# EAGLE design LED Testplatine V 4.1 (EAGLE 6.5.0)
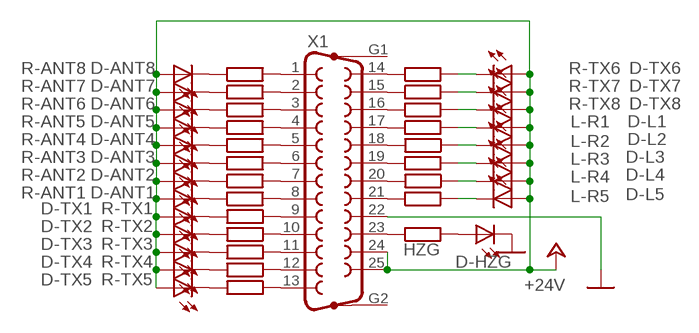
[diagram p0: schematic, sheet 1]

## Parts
D-ANT1  LEDCHIPLED_1206  [CHIPLED_1206]
D-ANT2  LEDCHIPLED_1206  [CHIPLED_1206]
D-ANT3  LEDCHIPLED_1206  [CHIPLED_1206]
D-ANT4  LEDCHIPLED_1206  [CHIPLED_1206]
D-ANT5  LEDCHIPLED_1206  [CHIPLED_1206]
D-ANT6  LEDCHIPLED_1206  [CHIPLED_1206]
D-ANT7  LEDCHIPLED_1206  [CHIPLED_1206]
D-ANT8  LEDCHIPLED_1206  [CHIPLED_1206]
D-HZG  LEDCHIPLED_1206  [CHIPLED_1206]
D-L1  LEDCHIPLED_1206  [CHIPLED_1206]
D-L2  LEDCHIPLED_1206  [CHIPLED_1206]
D-L3  LEDCHIPLED_1206  [CHIPLED_1206]
D-L4  LEDCHIPLED_1206  [CHIPLED_1206]
D-L5  LEDCHIPLED_1206  [CHIPLED_1206]
D-TX1  LEDCHIPLED_1206  [CHIPLED_1206]
D-TX2  LEDCHIPLED_1206  [CHIPLED_1206]
D-TX3  LEDCHIPLED_1206  [CHIPLED_1206]
D-TX4  LEDCHIPLED_1206  [CHIPLED_1206]
D-TX5  LEDCHIPLED_1206  [CHIPLED_1206]
D-TX6  LEDCHIPLED_1206  [CHIPLED_1206]
D-TX7  LEDCHIPLED_1206  [CHIPLED_1206]
D-TX8  LEDCHIPLED_1206  [CHIPLED_1206]
HZG  R-EU_R1206  [R1206]
L-R1  R-EU_R1206  [R1206]
L-R2  R-EU_R1206  [R1206]
L-R3  R-EU_R1206  [R1206]
L-R4  R-EU_R1206  [R1206]
L-R5  R-EU_R1206  [R1206]
R-ANT1  R-EU_R1206  [R1206]
R-ANT2  R-EU_R1206  [R1206]
R-ANT3  R-EU_R1206  [R1206]
R-ANT4  R-EU_R1206  [R1206]
R-ANT5  R-EU_R1206  [R1206]
R-ANT6  R-EU_R1206  [R1206]
R-ANT7  R-EU_R1206  [R1206]
R-ANT8  R-EU_R1206  [R1206]
R-TX1  R-EU_R1206  [R1206]
R-TX2  R-EU_R1206  [R1206]
R-TX3  R-EU_R1206  [R1206]
R-TX4  R-EU_R1206  [R1206]
R-TX5  R-EU_R1206  [R1206]
R-TX6  R-EU_R1206  [R1206]
R-TX7  R-EU_R1206  [R1206]
R-TX8  R-EU_R1206  [R1206]
X1  F25HP  [F25HP]

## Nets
+24V: D-ANT1.A D-ANT2.A D-ANT3.A D-ANT4.A D-ANT5.A D-ANT6.A D-ANT7.A D-ANT8.A D-L1.A D-L2.A D-L3.A D-L4.A D-L5.A D-TX1.A D-TX2.A D-TX3.A D-TX4.A D-TX5.A D-TX6.A D-TX7.A D-TX8.A X1.24 X1.25
GND: D-HZG.C X1.22
N$1: R-TX1.1 X1.9
N$2: R-TX2.1 X1.10
N$3: R-TX3.1 X1.11
N$4: R-TX4.1 X1.12
N$5: R-TX5.1 X1.13
N$6: L-R1.1 X1.17
N$7: R-TX6.1 X1.14
N$8: R-TX7.1 X1.15
N$9: R-TX8.1 X1.16
N$10: L-R2.2 X1.18
N$11: L-R3.1 X1.19
N$12: L-R4.2 X1.20
N$13: R-ANT8.2 X1.1
N$14: R-ANT7.2 X1.2
N$15: R-ANT6.2 X1.3
N$16: R-ANT5.2 X1.4
N$17: R-ANT4.2 X1.5
N$18: R-ANT3.2 X1.6
N$19: R-ANT2.2 X1.7
N$20: R-ANT1.2 X1.8
N$21: L-R5.1 X1.21
N$23: D-HZG.A HZG.2
N$24: D-L1.C L-R1.2
N$25: D-L3.C L-R3.2
N$26: D-L5.C L-R5.2
N$27: HZG.1 X1.23
N$28: D-L2.C L-R2.1
N$29: D-L4.C L-R4.1
N$31: D-TX1.C R-TX1.2
N$32: D-TX2.C R-TX2.2
N$33: D-TX3.C R-TX3.2
N$34: D-TX4.C R-TX4.2
N$35: D-ANT1.C R-ANT1.1
N$36: D-ANT2.C R-ANT2.1
N$37: D-ANT3.C R-ANT3.1
N$38: D-ANT4.C R-ANT4.1
N$39: D-TX5.C R-TX5.2
N$40: D-TX6.C R-TX6.2
N$41: D-TX7.C R-TX7.2
N$42: D-TX8.C R-TX8.2
N$43: D-ANT5.C R-ANT5.1
N$44: D-ANT6.C R-ANT6.1
N$45: D-ANT7.C R-ANT7.1
N$46: D-ANT8.C R-ANT8.1
Unconnected: X1.G1 X1.G2

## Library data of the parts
D-ANT1-D-ANT8 D-HZG D-L1-D-L5 D-TX1-D-TX8 = led:LED: LED
HZG L-R1-L-R5 R-ANT1-R-ANT8 R-TX1-R-TX8 = rcl:R-EU_: RESISTOR, European symbol
X1 = con-subd:F25HP: SUB-D; OC_FARNELL: unknown; OC_NEWARK: unknown

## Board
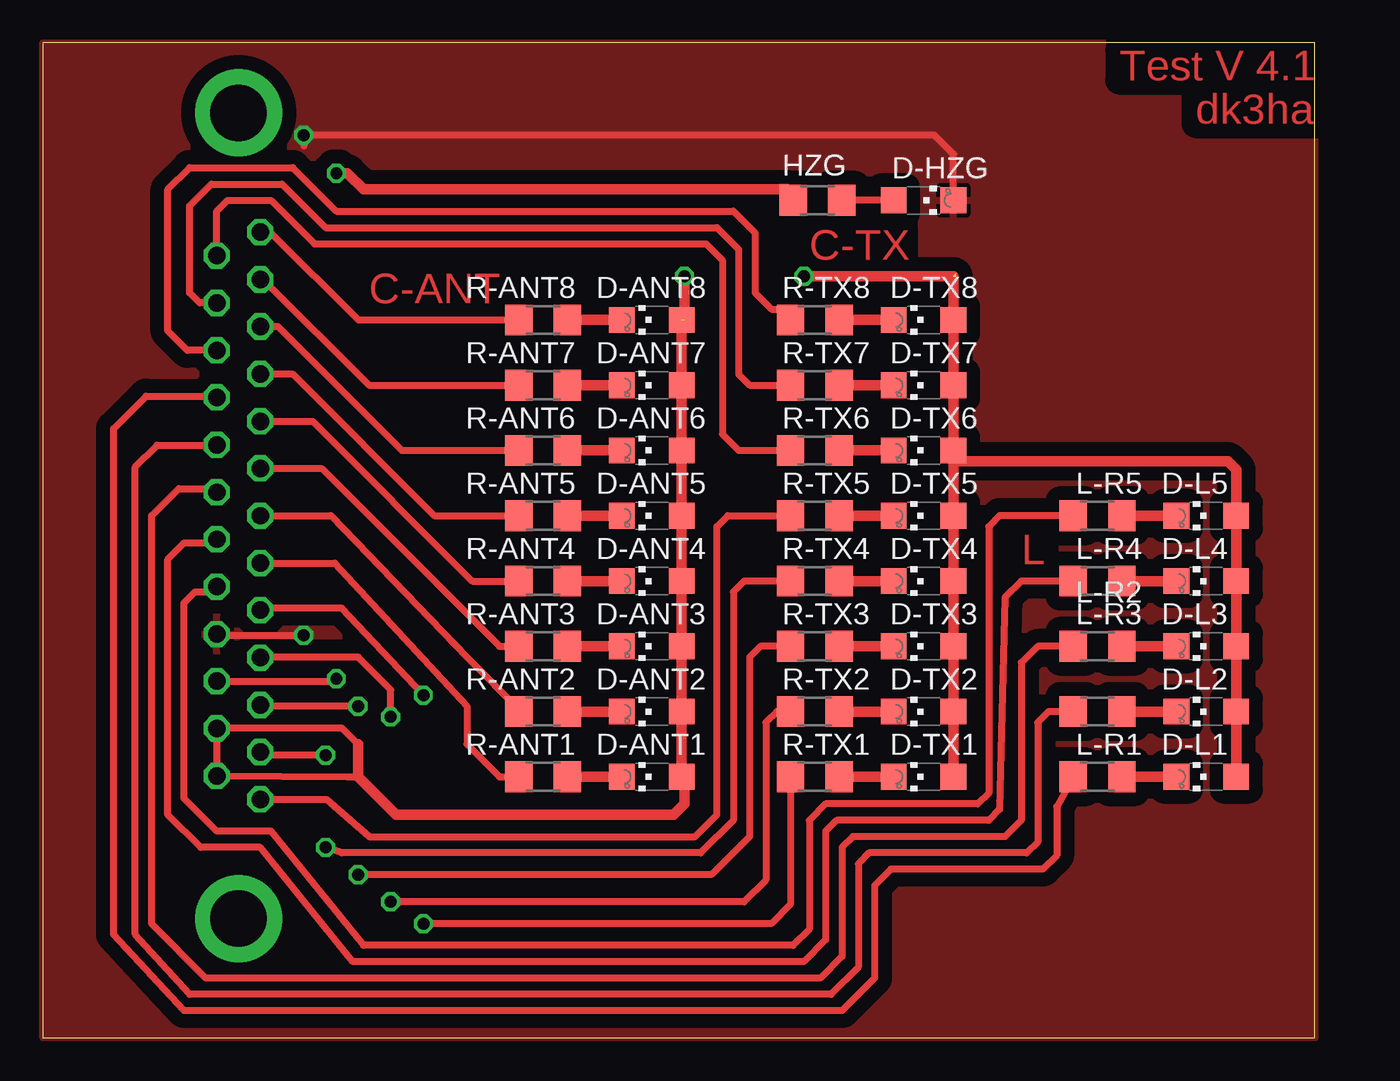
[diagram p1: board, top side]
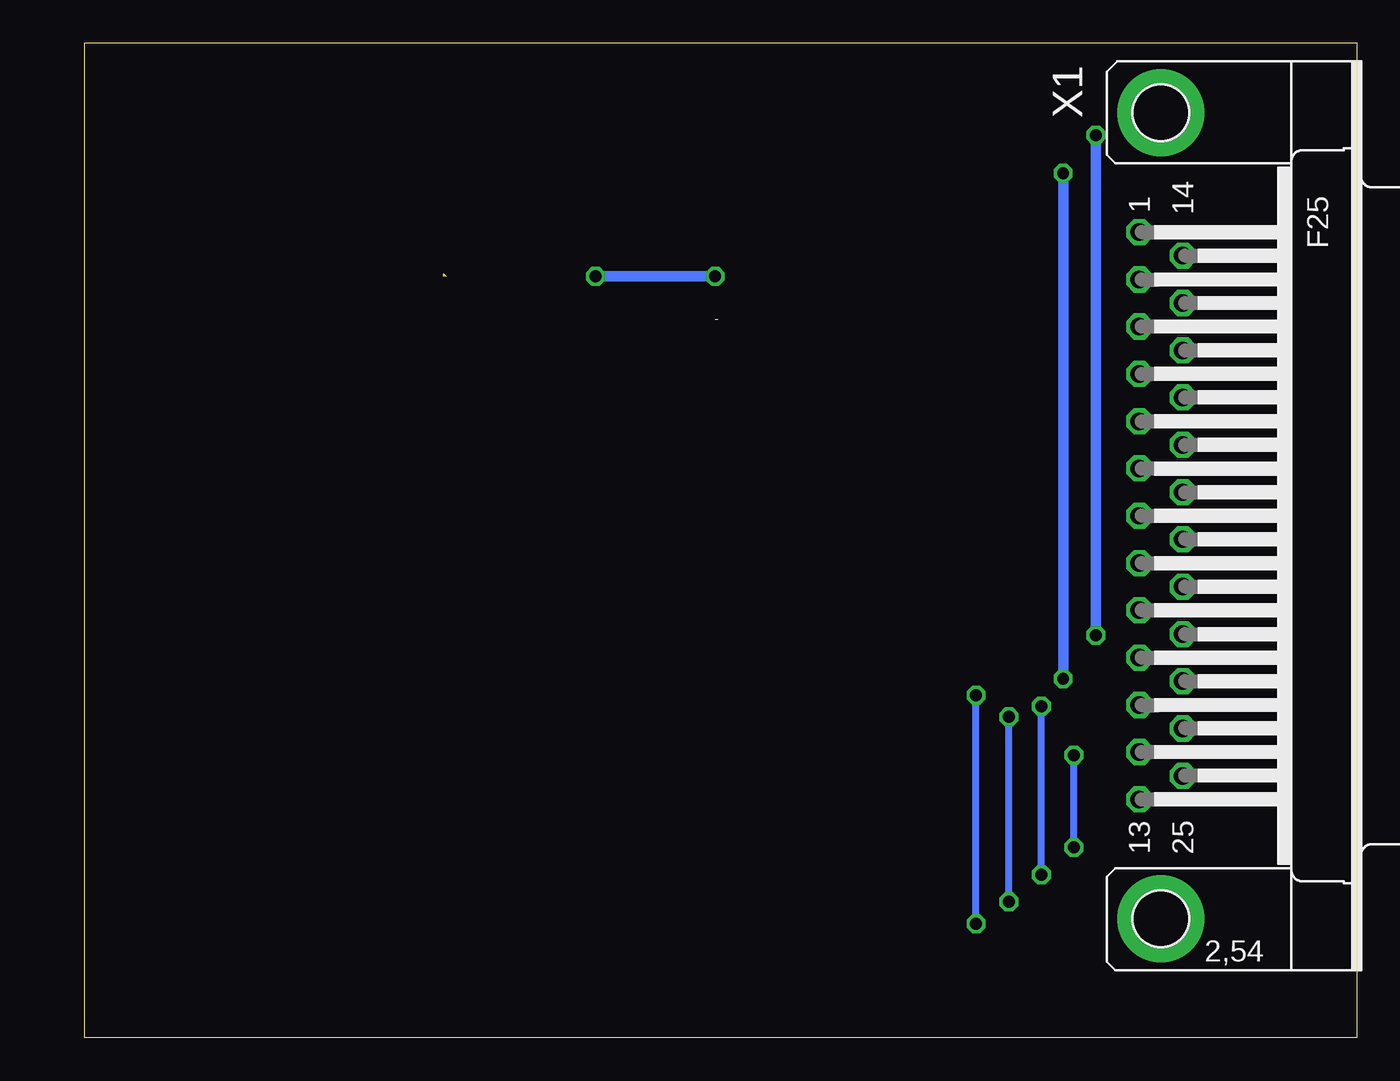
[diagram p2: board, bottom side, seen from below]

Size 74.28 x 58.09 mm. Coordinates in mm from the lower left corner, seen from the top.
Outline: 0,0 74.28,0 74.28,58.09 0,58.09 0,0
Copper layers (1*16): Top 0.035mm / dielectric 1.5mm / Bottom 0.035mm
Design rules "default *": minimum track width 10mil, minimum drill 24mil, track to track 8mil, track to pad 8mil, pad to pad 8mil, via to via 8mil, smd to smd 8mil, copper to edge 0mil, drill to drill 8mil, minimum pad ring 10mil, minimum via ring 8mil, stop-mask expansion 4mil, vias tented up to drill 0mil, thermal gap 10mil

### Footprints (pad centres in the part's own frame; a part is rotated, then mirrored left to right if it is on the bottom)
CHIPLED_1206 = smd 1.5 x 1.5: A 0,-1.75; C 0,1.75
R1206 = smd 1.6 x 1.803: 1 -1.422,0; 2 1.422,0
F25HP = drill 1.016 octagon: 1 -16.561,-1.27; 2 -13.792,-1.27; 3 -11.049,-1.27; 4 -8.28,-1.27; 5 -5.512,-1.27; 6 -2.769,-1.27; 7 0,-1.27; 8 2.769,-1.27; 9 5.512,-1.27; 10 8.28,-1.27; 11 11.049,-1.27; 12 13.792,-1.27; 13 16.561,-1.27; 14 -15.189,1.27; 15 -12.421,1.27; 16 -9.652,1.27; 17 -6.909,1.27; 18 -4.14,1.27; 19 -1.372,1.27; 20 1.372,1.27; 21 4.14,1.27; 22 6.909,1.27; 23 9.652,1.27; 24 12.421,1.27; 25 15.189,1.27 | drill 3.302 pad 5.08: G1 -23.52,0; G2 23.52,0

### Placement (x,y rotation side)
D-ANT1  35.56,15.24 90 top
D-ANT2  35.56,19.05 90 top
D-ANT3  35.56,22.86 90 top
D-ANT4  35.56,26.67 90 top
D-ANT5  35.56,30.48 90 top
D-ANT6  35.56,34.29 90 top
D-ANT7  35.56,38.1 90 top
D-ANT8  35.56,41.91 90 top
D-HZG  51.44,48.9 270 top
D-L1  67.94,15.24 90 top
D-L2  67.94,19.05 90 top
D-L3  67.94,22.86 90 top
D-L4  67.94,26.67 90 top
D-L5  67.94,30.48 90 top
D-TX1  51.44,15.24 90 top
D-TX2  51.44,19.05 90 top
D-TX3  51.44,22.86 90 top
D-TX4  51.44,26.67 90 top
D-TX5  51.44,30.48 90 top
D-TX6  51.44,34.29 90 top
D-TX7  51.44,38.1 90 top
D-TX8  51.44,41.91 90 top
HZG  45.24,48.9 0 top
L-R1  61.59,15.24 0 top
L-R2  61.59,19.05 180 top
L-R3  61.59,22.86 0 top
L-R4  61.59,26.67 180 top
L-R5  61.59,30.48 0 top
R-ANT1  29.21,15.24 180 top
R-ANT2  29.21,19.05 180 top
R-ANT3  29.21,22.86 180 top
R-ANT4  29.21,26.67 180 top
R-ANT5  29.21,30.48 180 top
R-ANT6  29.21,34.29 180 top
R-ANT7  29.21,38.1 180 top
R-ANT8  29.21,41.91 180 top
R-TX1  45.09,15.24 0 top
R-TX2  45.09,19.05 0 top
R-TX3  45.09,22.86 0 top
R-TX4  45.09,26.67 0 top
R-TX5  45.09,30.48 0 top
R-TX6  45.09,34.29 0 top
R-TX7  45.09,38.1 0 top
R-TX8  45.09,41.91 0 top
X1  11.43,30.48 270 bottom

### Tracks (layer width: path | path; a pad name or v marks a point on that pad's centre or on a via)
+24V  (via drill 0.7)  (4 unrouted)
  Top 0.406: X1.24 X1.25 17.78,15.24 18.41,15.24 | 37.47,15.09 D-ANT1.A | 10.16,18.1 17.46,18.1 18.41,17.14
  Top 0.61: D-ANT8.A D-ANT7.A D-ANT6.A D-ANT5.A D-ANT4.A D-ANT3.A D-ANT2.A D-ANT1.A | 53.19,33.66 D-TX6.A D-TX7.A D-TX8.A 53.19,44.45 v44.45,44.45 | 53.19,33.66 D-TX5.A D-TX4.A D-TX3.A D-TX2.A D-TX1.A | D-L1.A D-L2.A D-L3.A D-L4.A D-L5.A 69.69,33.17 69.22,33.66 53.19,33.66 | 37.47,15.09 37.47,13.65 36.83,13.02 20.64,13.02 18.41,15.24 18.41,17.14 | 37.47,41.91 v37.47,44.45
  Bottom 0.61: v37.47,44.45 v44.45,44.45
GND  (via drill 0.7)
  Top 0.406: v15.24,23.49 10.24,23.49 X1.22 | 15.24,52.07 v15.24,52.71 52.07,52.71 53.19,51.59 D-HZG.C
  Bottom 0.61: v15.24,23.49 v15.24,52.71
  pour Top (isolate 0.813): 0,58.1 74.3,58.1 74.3,0 0,0
N$1  (via drill 0.7)
  Top 0.406: R-TX1.1 43.66,7.79 42.55,6.67 v22.23,6.67 | v22.23,20 17.46,25.08 12.81,25.08 X1.9
  Bottom 0.406: v22.23,6.67 v22.23,20
N$2  (via drill 0.7)
  Top 0.406: R-TX2.1 42.86,19.05 42.23,18.41 42.23,9.21 40.96,7.94 v20.32,7.94 | v20.32,18.73 20.32,20.32 18.41,22.22 12.72,22.22 X1.10
  Bottom 0.406: v20.32,7.94 v20.32,18.73
N$3  (via drill 0.7)
  Top 0.406: R-TX3.1 41.91,22.86 41.27,22.22 41.27,11.75 39.05,9.53 v18.41,9.53 | v18.41,19.37 12.76,19.37 X1.11
  Bottom 0.406: v18.41,9.53 v18.41,19.37
N$4  (via drill 0.7)
  Top 0.406: R-TX4.1 40.96,26.67 40.32,26.04 40.32,12.7 38.42,10.79 17.46,10.79 v16.51,11.11 | v16.51,16.51 12.88,16.51 X1.12
  Bottom 0.406: v16.51,11.11 v16.51,16.51
N$5
  Top 0.406: X1.13 16.56,13.92 19.05,11.75 38.1,11.75 39.37,13.02 39.37,29.84 40.01,30.48 R-TX5.1
N$6
  Top 0.406: L-R1.1 59.22,13.5 59.22,10.64 58.42,9.84 49.53,9.84 48.58,8.89 48.58,3.49 46.67,1.59 8.26,1.59 4.13,6.03 4.13,35.56 6.03,37.47 10.08,37.47 X1.17
N$7
  Top 0.406: X1.14 10.16,48.26 10.79,48.9 13.34,48.9 15.88,46.36 38.73,46.36 39.69,45.4 39.69,35.24 40.64,34.29 R-TX6.1
N$8
  Top 0.406: X1.15 9.17,42.9 8.57,43.5 8.57,48.58 9.84,49.85 13.97,49.85 16.51,47.31 39.37,47.31 40.64,46.04 40.64,38.73 41.27,38.1 R-TX7.1
N$9
  Top 0.406: X1.16 8.45,40.13 7.3,41.28 7.3,49.53 8.57,50.8 14.61,50.8 17.14,48.26 40.32,48.26 41.59,46.99 41.59,43.5 42.55,42.55 43.81,42.55 R-TX8.1
N$10
  Top 0.406: L-R2.2 58.74,19.05 58.1,18.41 58.1,11.43 57.47,10.79 48.26,10.79 47.62,10.16 47.62,4.13 46.04,2.54 8.57,2.54 5.4,6.03 5.4,33.34 6.67,34.61 10.15,34.61 X1.18
N$11
  Top 0.406: L-R3.1 58.1,22.86 57.15,21.91 57.15,12.7 56.2,11.75 47.31,11.75 46.67,11.11 46.67,4.76 45.4,3.49 9.53,3.49 6.35,6.67 6.35,30.48 7.94,32.07 9.94,32.07 X1.19
N$12
  Top 0.406: L-R4.2 57.15,26.67 56.2,25.72 55.88,13.34 55.24,12.7 46.35,12.7 45.72,12.07 45.72,5.71 44.45,4.45 18.1,4.45 12.7,11.11 9.21,11.11 7.3,13.02 7.3,27.94 8.26,28.89 9.94,28.89 X1.20
N$13
  Top 0.406: X1.1 13.28,47.04 18.41,41.91 R-ANT8.2
N$14
  Top 0.406: X1.2 12.88,44.27 19.05,38.1 R-ANT7.2
N$15
  Top 0.406: X1.3 13.72,41.53 20.95,34.29 R-ANT6.2
N$16
  Top 0.406: X1.4 14.58,38.76 22.86,30.48 R-ANT5.2
N$17
  Top 0.406: X1.5 15.76,35.99 25.08,26.67 R-ANT4.2
N$18
  Top 0.406: X1.6 16.28,33.25 26.67,22.86 R-ANT3.2
N$19
  Top 0.406: X1.7 16.83,30.48 24.77,22.22 27.94,19.05 R-ANT2.2
N$20
  Top 0.406: X1.8 17.06,27.71 24.77,19.37 24.77,17.14 26.67,15.24 R-ANT1.2 27.94,15.24
N$21
  Top 0.406: L-R5.1 55.88,30.48 55.24,29.84 55.24,14.29 54.61,13.65 45.72,13.65 44.77,12.7 44.77,6.35 43.81,5.4 18.73,5.4 13.34,12.07 10.16,12.07 8.26,13.97 8.26,25.4 8.89,26.04 9.86,26.04 X1.21
N$23
  Top 0.406: D-HZG.A HZG.2
N$24
  Top 0.61: L-R1.2 D-L1.C
N$25
  Top 0.61: L-R3.2 D-L3.C
N$26
  Top 0.61: L-R5.2 D-L5.C
N$27  (via drill 0.7)
  Top 0.406: X1.23 17.02,20.83 v17.14,20.95
  Top 0.61: v17.14,50.48 17.78,50.48 18.73,49.53 43.5,49.53 HZG.1
  Bottom 0.61: v17.14,20.95 v17.14,50.48
N$28
  Top 0.61: L-R2.1 D-L2.C
N$29
  Top 0.61: L-R4.1 D-L4.C
N$31
  Top 0.61: R-TX1.2 D-TX1.C
N$32
  Top 0.61: R-TX2.2 D-TX2.C
N$33
  Top 0.61: R-TX3.2 D-TX3.C
N$34
  Top 0.61: R-TX4.2 D-TX4.C
N$35
  Top 0.61: R-ANT1.1 D-ANT1.C
N$36
  Top 0.61: R-ANT2.1 D-ANT2.C
N$37
  Top 0.61: R-ANT3.1 D-ANT3.C
N$38
  Top 0.61: R-ANT4.1 D-ANT4.C
N$39
  Top 0.61: R-TX5.2 D-TX5.C
N$40
  Top 0.61: R-TX6.2 D-TX6.C
N$41
  Top 0.61: R-TX7.2 D-TX7.C
N$42
  Top 0.61: R-TX8.2 D-TX8.C
N$43
  Top 0.61: R-ANT5.1 D-ANT5.C
N$44
  Top 0.61: R-ANT6.1 D-ANT6.C
N$45
  Top 0.61: R-ANT7.1 D-ANT7.C
N$46
  Top 0.61: R-ANT8.1 D-ANT8.C

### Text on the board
Top: Test V 4.1 | dk3ha | C-TX | C-ANT | L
